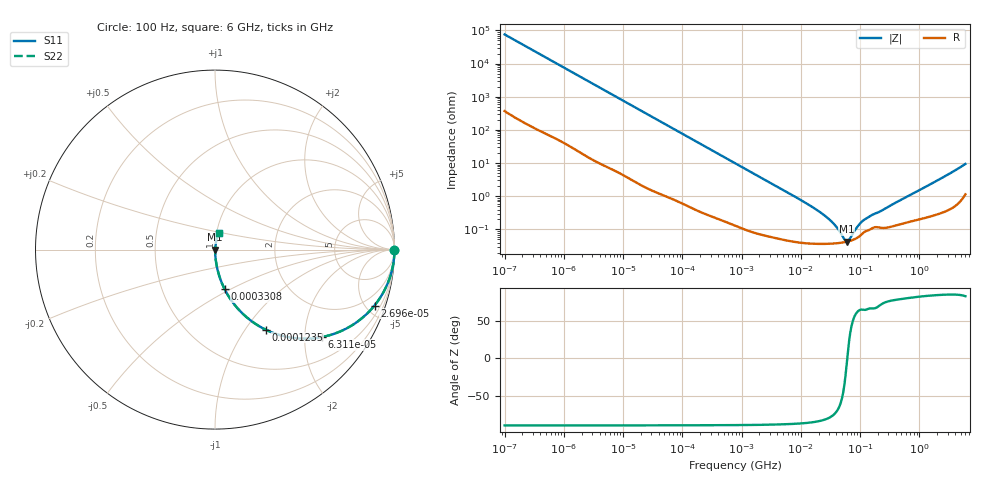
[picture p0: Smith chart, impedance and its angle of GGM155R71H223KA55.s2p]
!Murata Part Number: GGM155R71H223KA55
!These Parameters are Measured in Series Mode Connection
!Data Generated on Mar 13, 2026
!  o--ll--o
!Port1  Port2
!  o------o
!Operation Temp=25[degC], DC Bias Voltage=0[V]
!Freq. Start=100[Hz] Stop=6[GHz] 401[Steps]
# Hz S RI R 50
!Freq.(Hz) S11(Real) S11(Imag) S21(Real) S21(Imag) S12(Real) S12(Imag) S22(Real) S22(Imag)
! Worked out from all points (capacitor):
!   401 points, 100 Hz to 6 GHz, reference 50 ohm
!   read as one part in series: C = 21.1 nF near 109 Hz
!   lowest |Z| = 43 mohm at 59.6 MHz (marker M1)
!   series resonance near 60.81 MHz, so ESL is about 320 pH
!   S11 on the Smith chart (normalised r, x): 100 Hz: open; 26.96 kHz: 1.03, -5.69; 63.12 kHz: 1.02, -2.44; 123.5 kHz: 1.01, -1.25; 330.8 kHz: 1.00, -0.47; 6 GHz: 1.02, +0.19
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100  1 -0.00133  8.3e-06 0.00133  8.3e-06 0.00133  1 -0.00133
2008  0.9992 -0.0264  0.000831 0.0264  0.000831 0.0264  0.9992 -0.0264
8801  0.9863 -0.1135  0.0137 0.1135  0.0137 0.1135  0.9863 -0.1135
26957  0.8887 -0.3117  0.1113 0.3117  0.1113 0.3117  0.8887 -0.3117
40335  0.7823 -0.4095  0.2177 0.4095  0.2177 0.4095  0.7823 -0.4095
63115  0.5971 -0.4869  0.4029 0.4869  0.4029 0.4869  0.5971 -0.4869
123542  0.2824 -0.4462  0.7176 0.4462  0.7176 0.4462  0.2824 -0.4462
193316  0.1402 -0.3429  0.8598 0.3429  0.8598 0.3429  0.1402 -0.3429
330837  0.0541 -0.2212  0.9459 0.2212  0.9459 0.2212  0.0541 -0.2212
774597  0.0113 -0.0994  0.9887 0.0994  0.9887 0.0994  0.0113 -0.0994
2481164  0.00165 -0.0315  0.9984 0.0315  0.9984 0.0315  0.00165 -0.0315
1.555665e7  0.000396 -0.00477  0.9996 0.00477  0.9996 0.00477  0.000396 -0.00477
3.330331e7  0.000377 -0.00167  0.9996 0.00167  0.9996 0.00167  0.000377 -0.00167
4.165952e7  0.000387 -0.00101  0.9996 0.00101  0.9996 0.00101  0.000387 -0.00101
5.449875e7  0.000413 -0.000287  0.9996 0.000287  0.9996 0.000287  0.000413 -0.000287
5.960426e7  0.000427 -5.21e-05  0.9996 5.21e-05  0.9996 5.21e-05  0.000427 -5.21e-05
6.518806e7  0.000444 0.000183  0.9996 -0.000183  0.9996 -0.000183  0.000444 0.000183
8.918374e7  0.000558 0.00104  0.9994 -0.00104  0.9994 -0.00104  0.000558 0.00104
1.115611e8  0.000776 0.00166  0.9992 -0.00166  0.9992 -0.00166  0.000776 0.00166
3.124326e8  0.0012 0.00491  0.9988 -0.00491  0.9988 -0.00491  0.0012 0.00491
1.95892e9  0.00363 0.0288  0.9964 -0.0288  0.9964 -0.0288  0.00363 0.0288
6e9  0.0198 0.0911  0.9802 -0.0911  0.9802 -0.0911  0.0198 0.0911
